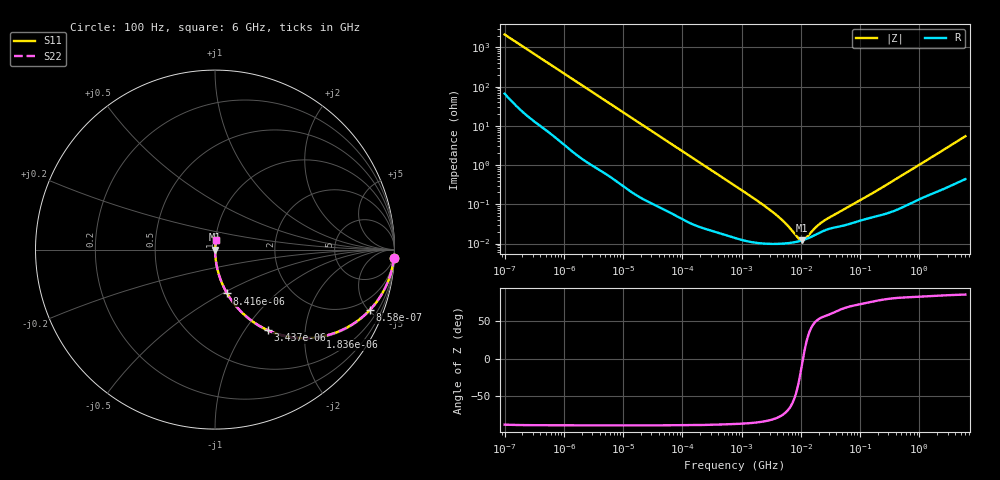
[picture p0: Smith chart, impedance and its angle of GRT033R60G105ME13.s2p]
!Murata Part Number: GRT033R60G105ME13
!These Parameters are Measured in Series Mode Connection
!Data Generated on Jun 19, 2026
!  o--ll--o
!Port1  Port2
!  o------o
!Operation Temp=25[degC], DC Bias Voltage=0[V]
!Freq. Start=100[Hz] Stop=6[GHz] 401[Steps]
# Hz S RI R 50
!Freq.(Hz) S11(Real) S11(Imag) S21(Real) S21(Imag) S12(Real) S12(Imag) S22(Real) S22(Imag)
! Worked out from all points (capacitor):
!   401 points, 100 Hz to 6 GHz, reference 50 ohm
!   read as one part in series: C = 744 nF near 109 Hz
!   lowest |Z| = 12.1 mohm at 10.4 MHz (marker M1)
!   series resonance near 10.91 MHz, so ESL is about 290 pH
!   S11 on the Smith chart (normalised r, x): 100 Hz: 2, -43; 858 Hz: 1.08, -5.07; 1.836 kHz: 1.03, -2.38; 3.437 kHz: 1.02, -1.28; 8.416 kHz: 1.01, -0.53; 6 GHz: 1.01, +0.11
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100  0.9964 -0.0467  0.00364 0.0467  0.00364 0.0467  0.9964 -0.0467
320  0.9757 -0.1448  0.0243 0.1448  0.0243 0.1448  0.9757 -0.1448
548  0.936 -0.236  0.064 0.236  0.064 0.236  0.936 -0.236
858  0.8614 -0.3376  0.1386 0.3376  0.1386 0.3376  0.8614 -0.3376
1227  0.7564 -0.4221  0.2436 0.4221  0.2436 0.4221  0.7564 -0.4221
1836  0.5854 -0.486  0.4146 0.486  0.4146 0.486  0.5854 -0.486
2008  0.5423 -0.4916  0.4577 0.4916  0.4577 0.4916  0.5423 -0.4916
3437  0.2926 -0.4483  0.7074 0.4483  0.7074 0.4483  0.2926 -0.4483
5378  0.1474 -0.3477  0.8526 0.3477  0.8526 0.3477  0.1474 -0.3477
8416  0.0676 -0.2445  0.9324 0.2445  0.9324 0.2445  0.0676 -0.2445
17227  0.018 -0.1267  0.982 0.1267  0.982 0.1267  0.018 -0.1267
40335  0.00392 -0.0553  0.9961 0.0553  0.9961 0.0553  0.00392 -0.0553
774597  0.000147 -0.00297  0.9999 0.00297  0.9999 0.00297  0.000147 -0.00297
3712478  9.82e-05 -0.000554  0.9999 0.000554  0.9999 0.000554  9.82e-05 -0.000554
5554849  0.000101 -0.000309  0.9999 0.000309  0.9999 0.000309  0.000101 -0.000309
9090158  0.000113 -7.64e-05  0.9999 7.64e-05  0.9999 7.64e-05  0.000113 -7.64e-05
1.039699e7  0.00012 -1.98e-05  0.9999 1.98e-05  0.9999 1.98e-05  0.00012 -1.98e-05
1.189169e7  0.000128 3.54e-05  0.9999 -3.54e-05  0.9999 -3.54e-05  0.000128 3.54e-05
1.555665e7  0.000152 0.000143  0.9998 -0.000143  0.9998 -0.000143  0.000152 0.000143
2.662322e7  0.000223 0.000345  0.9998 -0.000345  0.9998 -0.000345  0.000223 0.000345
3.124326e8  0.000625 0.00341  0.9994 -0.00341  0.9994 -0.00341  0.000625 0.00341
6e9  0.00725 0.0536  0.9927 -0.0536  0.9927 -0.0536  0.00725 0.0536
